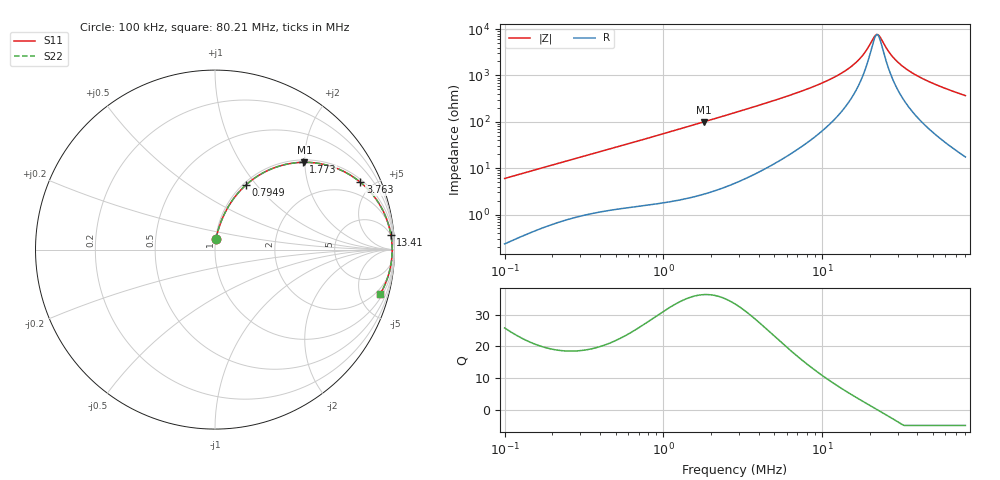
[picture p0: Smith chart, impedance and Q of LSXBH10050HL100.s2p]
! LSXBH10050HL100  S-PARAMETER MODEL  ( General Type )
! Model Generated by TAIYO YUDEN Corporation (http://www.ty-top.com)
! Version 3.0
! TAIYO YUDEN Control No. 180118NI43SB-FBB
! Copyright(c) 2007 TAIYO YUDEN CO.,LTD. All Rights Reserved.
! Product Description (link to TY-COMPAS)
! https://ds.yuden.co.jp/TYCOMPAS/or/detail?pn=LSXBH10050HL100M&u=M
! Products Name : Inductors
! Characteristics :
!  Inductance : 10 uH , SRF(min) : 15 MHz , DC Resistance(max) : 0.0325 Ohm
!  Rated Current : Saturation :4700 mA , Temp Rise : 4100 mA (40 degC)
!  Case Size : 10.0 x 9.8 / 0.394 x 0.386 [mm/inch] , Thickness : 5 / 0.197 [mm/inch]
!  (Conditions: Temperature = 25 degC , DC Bias Current/Voltage = 0A / 0V)
! External Node Assignments :
!  1  o---GGG---o  2
! GND o---------o GND
! Frequency Range : 0.1MHz  -  80.209071MHz  [ 402 STEP ]
# MHz S RI R 50
! Freq[MHz].  S11 Real  S11 Imag  S21 Real  S21 Imag  S12 Real  S12 Imag  S22 Real  S22 Imag
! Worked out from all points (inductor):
!   401 points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, 100 kHz to 80.21 MHz, reference 50 ohm
!   read as one part in series: L = 9.45 uH near 103.4 kHz
!   highest Q = 36.3 at 1.803 MHz (marker M1), where L = 8.79 uH
!   self-resonance near 22.14 MHz
!   S11 on the Smith chart (normalised r, x): 100 kHz: 1.00, +0.12; 794.9 kHz: 1.03, +0.88; 1.773 MHz: 1.05, +1.96; 3.763 MHz: 1.15, +4.24; 13.41 MHz: 4, +23; 80.21 MHz: 1.35, -7.32
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0.1  0.00586 0.0593  0.9941 -0.0593  0.9941 -0.0593  0.00586 0.0593
0.306519  0.0382 0.1668  0.9618 -0.1668  0.9618 -0.1668  0.0382 0.1668
0.523354  0.0889 0.263  0.9111 -0.263  0.9111 -0.263  0.0889 0.263
0.794894  0.1712 0.3591  0.8288 -0.3591  0.8288 -0.3591  0.1712 0.3591
0.939539  0.2201 0.398  0.7799 -0.398  0.7799 -0.398  0.2201 0.398
1.773438  0.4902 0.4863  0.5098 -0.4863  0.5098 -0.4863  0.4902 0.4863
1.803336  0.4984 0.4864  0.5016 -0.4864  0.5016 -0.4864  0.4984 0.4864
2.832121  0.708 0.44  0.292 -0.44  0.292 -0.44  0.708 0.44
3.763061  0.8101 0.3752  0.1899 -0.3752  0.1899 -0.3752  0.8101 0.3752
5.527568  0.9017 0.2752  0.0983 -0.2752  0.0983 -0.2752  0.9017 0.2752
8.680988  0.957 0.1683  0.043 -0.1683  0.043 -0.1683  0.957 0.1683
13.40737  0.9798 0.0839  0.0202 -0.0839  0.0202 -0.0839  0.9798 0.0839
17.22868  0.9853 0.0413  0.0147 -0.0413  0.0147 -0.0413  0.9853 0.0413
19.04651  0.9864 0.025  0.0136 -0.025  0.0136 -0.025  0.9864 0.025
21.41112  0.9871 0.00623  0.0129 -0.00623  0.0129 -0.00623  0.9871 0.00623
22.13913  0.9871 0.000887  0.0129 -0.000887  0.0129 -0.000887  0.9871 0.000887
23.27781  0.9871 -0.00713  0.0129 0.00713  0.0129 0.00713  0.9871 -0.00713
26.60888  0.9863 -0.0286  0.0137 0.0286  0.0137 0.0286  0.9863 -0.0286
31.45084  0.984 -0.0561  0.016 0.0561  0.016 0.0561  0.984 -0.0561
39.08584  0.9782 -0.0939  0.0218 0.0939  0.0218 0.0939  0.9782 -0.0939
53.69948  0.9621 -0.1555  0.0379 0.1555  0.0379 0.1555  0.9621 -0.1555
80.20907  0.9206 -0.2477  0.0794 0.2477  0.0794 0.2477  0.9206 -0.2477
